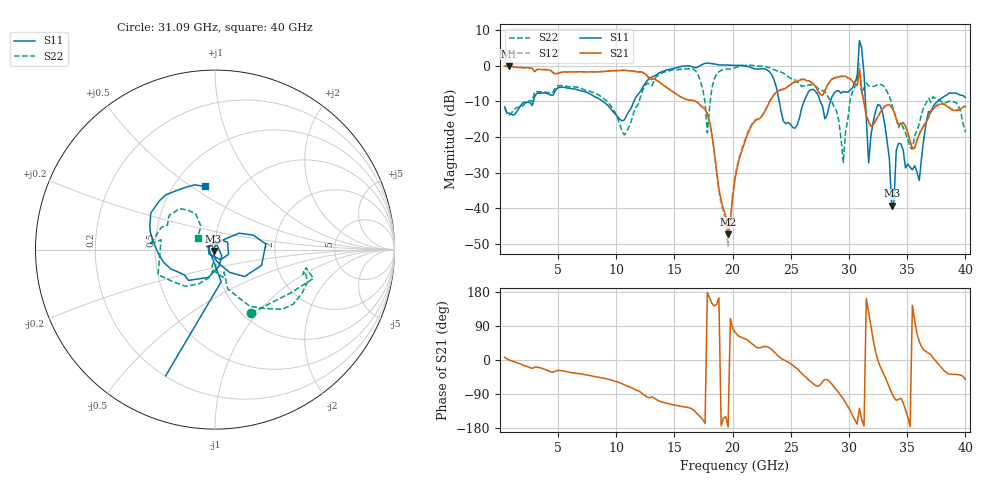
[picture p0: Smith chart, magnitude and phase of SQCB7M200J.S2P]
! Network Analyzer HP8722ES.07.66: Jul 25, 2000 Serial No. US39175408
! 27 Oct 2004  08:24:31
! Frequency  S11  S21  S12  S22
# HZ  S  DB R  50
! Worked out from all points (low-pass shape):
!   201 points, 400 MHz to 40 GHz, reference 50 ohm
!   highest |S21| = -0.15 dB at 796 MHz (marker M1); lowest = -47.3 dB at 19.61 GHz (marker M2)
!   |S21| within 3 dB of the highest: start of sweep to 12.71 GHz; 29.19 GHz to 29.75 GHz (565.1 MHz wide, 1.92 % of centre)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
!   lowest |S11| = -39.3 dB at 33.66 GHz (marker M3), VSWR 1.02, Z = 49.2 - j0.681 ohm
!   |S11| at or under -10 dB: start of sweep to 2.873 GHz; 8.829 GHz to 11.52 GHz (2.696 GHz wide, 26.5 % of centre); 31.41 GHz to 37.63 GHz (6.22 GHz wide, 18 % of centre)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
!   |S22| runs from -27.2 to 0.1 dB; largest |S21 - S12| = 0.27
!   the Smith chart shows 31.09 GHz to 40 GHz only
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4e8  -11.57 -85.0  -0.17 7.2  -0.07 8.8  -11.92 -81.0
7.96e8  -13.34 -82.2  -0.15 -0.1  -0.38 0.8  -13.87 -92.8
7.132e9  -7.24 -115.3  -1.77 -37.5  -1.86 -38.2  -6.64 -124.3
1.0696e10  -15.26 -45.9  -1.34 -65.5  -1.35 -65.8  -19.46 -75.8
1.3666e10  -2.12 -18.2  -4.58 -108.2  -4.62 -108.1  -2.56 -26.6
1.6834e10  -0.62 -20.8  -10.07 -137.9  -10.09 -138.6  -1.57 -72.3
1.7824e10  0.69 -19.4  -13.50 178.2  -13.54 176.3  -18.86 -53.4
1.9606e10  0.15 -20.8  -47.28 -176.7  -50.66 155.0  -0.97 -22.7
2.02e10  0.07 -22.2  -31.81 73.5  -30.88 70.1  -0.61 -22.9
2.6932e10  -6.69 37.8  -5.13 -63.0  -5.18 -63.6  -5.61 -41.0
2.9506e10  -7.30 61.8  -3.07 -102.8  -3.11 -103.4  -27.19 -169.8
3.0694e10  -3.71 68.4  -5.64 -169.2  -5.63 -169.7  -2.54 73.8
3.0892e10  7.02 33.8  -1.36 -127.9  0.57 -137.5  -0.81 -149.0
3.109e10  4.76 -89.9  -7.10 -157.2  -7.24 -158.8  -7.81 -60.3
3.1684e10  -27.28 155.9  -15.81 126.3  -15.50 126.0  -5.72 -11.2
3.2476e10  -10.91 6.3  -14.38 -0.5  -14.57 0.9  -5.25 -18.9
3.3466e10  -26.07 -92.5  -11.01 -72.1  -10.99 -71.5  -8.58 -58.3
3.3664e10  -39.34 -140.1  -11.72 -86.2  -11.66 -85.7  -10.62 -64.2
3.4258e10  -21.83 29.9  -16.70 -103.7  -16.83 -102.6  -17.39 -67.9
3.604e10  -32.20 -9.8  -19.30 48.7  -19.02 48.7  -16.25 -99.5
3.6832e10  -12.89 -130.8  -14.67 18.3  -14.41 19.3  -9.20 -156.3
4e10  -8.95 99.1  -11.48 -51.3  -11.28 -50.7  -18.65 145.7
